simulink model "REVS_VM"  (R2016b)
settings: Solver=ode3  StartTime=REVS.sim_start_time_secs  StopTime=Inf  FixedStep=REVS.sim_step_time_secs  MaxStep=REVS.sim_step_time_secs  EnableMultiTasking=on
StopFcn:
  | postproc_datalog;
  | postproc_audit;
  | postproc_result;
model workspace (MATLAB code in the model file):
  other statements: REVS_setup_variants
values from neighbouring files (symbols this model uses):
  accessory = class_accessory_data    [class_test_data.m]
  battery = class_battery_data    [class_accessory_data.m]    (also in class_REVS_electric.m = class_REVS_battery)
  brake = struct(	'max_torque_Nm',[], 						'proportion_norm',1.0, 						'inertia_kgm2',0.0)    [class_REVS_drive_axle.m]
  engine = class_engine_data    [class_test_data.m]
  final_drive = struct(	'gear_ratio',[], 								'efficiency_norm',[], 								'inertia_kgm2',[] )    [class_REVS_drive_axle.m]
  gear = class_REVS_gearbox    [class_REVS_AT_transmission.m]
  tire = struct(	'radius_m',[], 						'rolling_resistance_coefficient',0, 						'vehicle_weight_norm',1.0,  						'wheel_slip_torque_Nm',[],  						'inertia_kgm2',0.0)    [class_REVS_drive_axle.m]
  torque_converter = class_REVS_torque_converter    [class_REVS_AT_transmission.m]
  transmission = class_transmission_data    [class_test_data.m]
  vehicle = class_vehicle_data    [class_test_data.m]
undefined symbols (not defined in the file or in its folder): alternator, ambient, controls, convert, DelayTimeSecs, drive_cycle, driver, electric, gear_strategy, InitialCondition, InitialValue, LoadSource, LookupStructure, MultiplyPosInputs, Normalize, NumPhases, REVS, SpeedSource, starter, tableshift, UpperSaturationLimit, Value, VerboseLevel, VerboseSignal
libraries: simulink x153
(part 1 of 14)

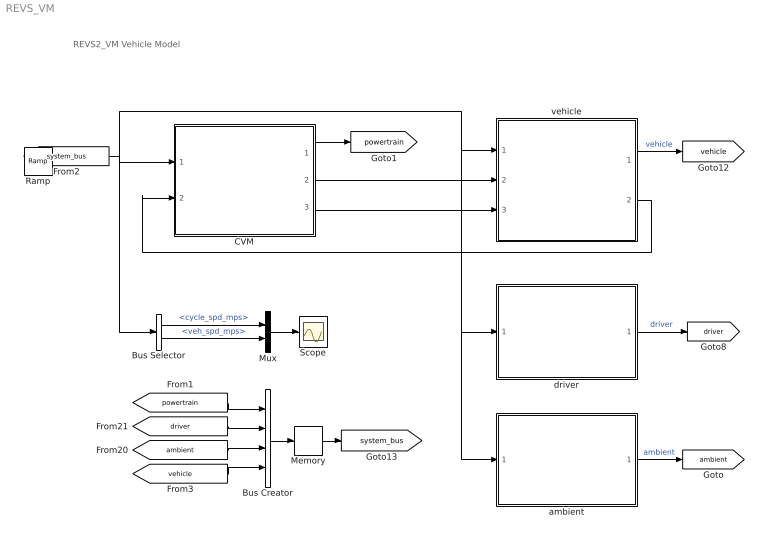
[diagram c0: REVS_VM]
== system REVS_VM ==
  note: REVS2_VM Vehicle Model
  Bus Creator : BusCreator  Inputs=4
  Bus Selector : BusSelector  OutputSignals=driver.cycle_spd_mps,vehicle.veh_spd_mps
  CVM : Subsystem  VariantControl=get_REVS_powertrain_type(REVS) == enum_powertrain_type.conventional
  Memory : Memory
  Mux : Mux  Inputs=2
  Scope : Scope
  ambient : Subsystem
  driver : Subsystem  VariantControl=variants_driver_MT
  vehicle : Subsystem
  Ramp : simulink/Sources/Ramp  IOType=siggen  slope=1  start=0  X0=0
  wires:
  vehicle/1(bus_out) -> [vehicle]  "vehicle"
  Bus Selector/1 -> Mux/1  "<cycle_spd_mps>"
  Bus Selector/2 -> Mux/2  "<veh_spd_mps>"
  Mux/1 -> Scope/1
  Bus Creator/1 -> Memory/1
  [driver] -> Bus Creator/2
  [ambient] -> Bus Creator/3
  Memory/1 -> [system_bus]
  [system_bus] -> CVM/1(system_bus), vehicle/1(system_bus), ambient/1(system_bus), driver/1(system_bus), Bus Selector/1
  [powertrain] -> Bus Creator/1
  [vehicle] -> Bus Creator/4
  vehicle/2(veh_spd_mps) -> CVM/2(veh_spd_mps)
  CVM/2(force_out_N) -> vehicle/2(force_in_N)
  CVM/3(mass_out_kg) -> vehicle/3(mass_in_kg)
  CVM/1(bus_out) -> [powertrain]
  ambient/1(bus_out) -> [ambient]  "ambient"
  driver/1(bus_out) -> [driver]  "driver"

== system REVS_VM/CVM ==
  note: ALPHA_CVM Conventional Vehicle Model
  system_bus : Inport
  veh_spd_mps : Inport  Port=2
  ALPHA CVM electric & accessories : Subsystem  VariantControl=variants_electric_ALPHA
  Bus Creator1 : BusCreator  Inputs=4
  CVM control : Subsystem
  automatic transmission system : Subsystem  VariantControl=get_REVS_transmission_type(transmission) == enum_transmission_type.automatic
  engine : Subsystem  Variant=on
  one axle drive : Subsystem  VariantControl=vehicle_driveline_type == enum_driveline_type.one_axle_drive
  bus_out : Outport
  force_out_N : Outport  Port=2
  mass_out_kg : Outport  Port=3
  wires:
  one axle drive/2(mass_out_kg) -> mass_out_kg/1
  one axle drive/1(force_out_N) -> force_out_N/1
  veh_spd_mps/1 -> one axle drive/4(spd_out_mps)
  system_bus/1 -> one axle drive/1(system_bus), automatic transmission system/1(system_bus), ALPHA CVM electric & accessories/1(system_bus), engine/1(system_bus), CVM control/1(system_bus)
  [trans] -> Bus Creator1/3
  [engine] -> Bus Creator1/2
  [control] -> Bus Creator1/1
  [electric] -> Bus Creator1/4
  Bus Creator1/1 -> bus_out/1  "powertrain"
  engine/2(eng_trq_Nm) -> automatic transmission system/2(trq_in_Nm)
  automatic transmission system/1(bus_out) -> [trans]
  engine/1(bus_out) -> [engine]
  automatic transmission system/2(trq_out_Nm) -> one axle drive/2(trq_in_Nm)
  ALPHA CVM electric & accessories/1(bus_out) -> [electric]
  automatic transmission system/3(iner_out_kgm2) -> one axle drive/3(iner_in_kgm2)
  one axle drive/3(spd_in_radps) -> automatic transmission system/4(spd_out_radps)
  ALPHA CVM electric & accessories/3(iner_out_kgm2) -> engine/3(acc_iner_kgm2)
  engine/3(eng_iner_kgm2) -> automatic transmission system/3(iner_in_kgm2)
  automatic transmission system/4(spd_in_radps) -> engine/4(eng_spd_radps), ALPHA CVM electric & accessories/2(spd_in_radps)
  ALPHA CVM electric & accessories/2(trq_out_Nm) -> engine/2(acc_trq_Nm)
  CVM control/1(bus_out) -> [control]

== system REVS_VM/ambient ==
  system_bus : Inport
  1-D Lookup Table : Lookup_n-D  NumberOfTableDimensions=1  BreakpointsForDimension1=drive_cycle.grade_dist_m  IndexSearchMethod=Linear search  BeginIndexSearchUsingPreviousIndexResult=on  Table=drive_cycle.grade_pct  ExtrapMethod=Clip  UseLastTableValue=on  RndMeth=Simplest
  Bus Creator : BusCreator  Inputs=2
  Bus Selector : BusSelector  OutputSignals=signal4.veh_dist_m
  Constant : Constant  Value=ambient.temperature_degC
  Time Logging : Subsystem
  datalog cycle grade : Subsystem
  bus_out : Outport
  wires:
  Constant/1 -> Bus Creator/2  "temp_degC"
  1-D Lookup Table/1 -> datalog cycle grade/1(Var), Bus Creator/1  "drive_cycle_grade_pct"
  Bus Creator/1 -> bus_out/1  "ambient"
  system_bus/1 -> Bus Selector/1
  Bus Selector/1 -> 1-D Lookup Table/1  "<veh_dist_m>"

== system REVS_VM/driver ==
  system_bus : Inport
  > 0 : Saturate  UpperLimit=Inf  LowerLimit=0
  Bus Creator1 : BusCreator  Inputs=8
  Compare To Zero : simulink/Logic and Bit Operations/Compare To Zero  relop=>  OutDataTypeStr=boolean
  Product : Product
  Product1 : Product
  closed loop driver : Subsystem
  cycle position : Subsystem
  datalog driver acl : Subsystem
  datalog driver brk : Subsystem
  drive cycle lookups : Subsystem
  bus_out : Outport
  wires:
  > 0/1 -> Bus Creator1/5  "cycle_spd_mps"
  drive cycle lookups/6(cycle_phase) -> Bus Creator1/7  "cycle_phase_num"
  drive cycle lookups/1(veh_spd_des_mps) -> closed loop driver/2(veh_spd_des_mps), > 0/1
  drive cycle lookups/2(future_veh_spd_des_mps) -> closed loop driver/3(future_veh_spd_des_mps)
  system_bus/1 -> cycle position/1(system_bus), closed loop driver/1(system_bus)
  Bus Creator1/1 -> bus_out/1  "driver"
  closed loop driver/1(acl_pedal_norm) -> Product/1
  closed loop driver/2(brk_pedal_norm) -> Product1/1
  drive cycle lookups/4(driver_key_pos) -> Bus Creator1/4  "driver_ign_keyon"
  Product/1 -> datalog driver acl/1(Var), Bus Creator1/1  "driver_acl_norm"
  Product1/1 -> datalog driver brk/1(Var), Bus Creator1/2  "driver_brk_norm"
  drive cycle lookups/3(driver_in_gear) -> Product/2, Product1/2, Bus Creator1/3  "driver_in_gear"
  cycle position/1(cycle_position_secs) -> Bus Creator1/8, drive cycle lookups/1(cycle_position_secs)  "cycle_pos_secs"
  drive cycle lookups/5(anticipate_veh_spd_des_mps) -> Compare To Zero/1
  Compare To Zero/1 -> Bus Creator1/6  "accel_anticipate_bool"

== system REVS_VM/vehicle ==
  system_bus : Inport
  force_in_N : Inport  Port=2
  mass_in_kg : Inport  Port=3
  Bus Creator : BusCreator  Inputs=2
  vehicle net force : Subsystem  VariantControl=vehicle_use_abc_roadload == true
  vehicle speed integrator : Subsystem
  bus_out : Outport
  veh_spd_mps : Outport  Port=2
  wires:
  Bus Creator/1 -> bus_out/1  "vehicle"
  system_bus/1 -> vehicle net force/1(system_bus), vehicle speed integrator/1(system_bus)
  force_in_N/1 -> vehicle net force/2(force_in_N)
  mass_in_kg/1 -> vehicle speed integrator/3(mass_in_kg)
  vehicle net force/1(force_out_N) -> vehicle speed integrator/2(force_out_N)
  vehicle speed integrator/1(veh_spd_mps) -> Bus Creator/1, veh_spd_mps/1, vehicle net force/3(chs_spd_mps)  "veh_spd_mps"
  vehicle speed integrator/2(veh_dist_m) -> Bus Creator/2  "veh_dist_m"

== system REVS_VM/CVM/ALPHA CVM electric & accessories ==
  system_bus : Inport
  spd_in_radps : Inport  Port=2
  Bus Creator : BusCreator  Inputs=2
  CVM accessories : Subsystem  VariantControl=variants_electric_ALPHA
  CVM electric : Subsystem  VariantControl=variants_electric_ALPHA
  Sum2 : Sum
  Sum6 : Sum
  bus_out : Outport
  trq_out_Nm : Outport  Port=2
  iner_out_kgm2 : Outport  Port=3
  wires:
  spd_in_radps/1 -> CVM accessories/2(spd_in_radps), CVM electric/2(spd_in_radps)
  Bus Creator/1 -> bus_out/1
  system_bus/1 -> CVM electric/1(system_bus), CVM accessories/1(system_bus)
  Sum6/1 -> iner_out_kgm2/1
  Sum2/1 -> trq_out_Nm/1
  CVM accessories/4(curr_out_A) -> CVM electric/3(curr_in_A)
  CVM electric/3(iner_out_kgm2) -> Sum6/1
  CVM electric/1(bus_out) -> Bus Creator/1  "elec"
  CVM accessories/1(bus_out) -> Bus Creator/2  "accy"
  CVM electric/4(volt_out_V) -> CVM accessories/3(voltage_V)
  CVM accessories/3(iner_out_kgm2) -> Sum6/2
  CVM accessories/2(trq_out_Nm) -> Sum2/2
  CVM electric/2(trq_out_Nm) -> Sum2/1

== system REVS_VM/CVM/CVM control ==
  system_bus : Inport
  Bus Creator : BusCreator  Inputs=1
  start stop logic : Subsystem
  bus_out : Outport
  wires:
  start stop logic/1(engine_on) -> Bus Creator/1  "ctrl_eng_on"
  system_bus/1 -> start stop logic/1(system_bus)
  Bus Creator/1 -> bus_out/1  "control"

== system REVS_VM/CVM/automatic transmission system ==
  system_bus : Inport
  trq_in_Nm : Inport  Port=2
  iner_in_kgm2 : Inport  Port=3
  spd_out_radps : Inport  Port=4
  Bus Creator : BusCreator  Inputs=4
  automatic trans control : Subsystem  VariantControl=variants_trans_control_default
  automatic transmission core : Subsystem  VariantControl=variants_trans_automatic
  result work : Subsystem
  thermal model : Subsystem  Variant=on
  to datalog : Subsystem
  to datalog1 : Subsystem
  to datalog2 : Subsystem
  torque converter : Subsystem
  bus_out : Outport
  trq_out_Nm : Outport  Port=2
  iner_out_kgm2 : Outport  Port=3
  spd_in_radps : Outport  Port=4
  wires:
  thermal model/1(thermal_bus) -> Bus Creator/2  "therm"
  automatic transmission core/4(spd_in_radps) -> torque converter/4(spd_out_radps)
  torque converter/4(spd_in_radps) -> spd_in_radps/1
  spd_out_radps/1 -> to datalog2/1(Var), result work/2(speed_radps), automatic transmission core/4(spd_out_radps)  "trans_spd_out_radps"
  torque converter/3(iner_out_kgm2) -> automatic transmission core/3(iner_in_kgm2)
  torque converter/2(trq_out_Nm) -> automatic transmission core/2(trq_in_Nm)
  iner_in_kgm2/1 -> torque converter/3(iner_in_kgm2)
  trq_in_Nm/1 -> torque converter/2(trq_in_Nm)
  automatic transmission core/3(iner_out_kgm2) -> iner_out_kgm2/1, to datalog1/1(Var), result work/3(upstream_iner_kgm2)
  automatic transmission core/2(trq_out_Nm) -> to datalog/1(Var), result work/1(torque_Nm), trq_out_Nm/1
  automatic transmission core/1(bus_out) -> Bus Creator/4  "core"
  automatic trans control/1(bus_out) -> Bus Creator/1  "ctrl"
  system_bus/1 -> automatic trans control/1(system_bus), thermal model/1(system_bus)
  Bus Creator/1 -> bus_out/1, torque converter/1(trans_bus), automatic transmission core/1(trans_bus)  "trans"
  torque converter/1(bus_out) -> Bus Creator/3  "trq_conv"

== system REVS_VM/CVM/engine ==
  note: 1) Only subsystems can be added as variant choices at this level 2) Blocks cannot be connected at this level as connectivity is automatically determined at simulation, based on the active variant
  system_bus : Inport
  acc_trq_Nm : Inport  Port=2
  acc_iner_kgm2 : Inport  Port=3
  eng_spd_radps : Inport  Port=4
  legacy engine : Subsystem  VariantControl=get_REVS_engine_model_type(engine) == enum_engine_model_type.legacy
  new engine : Subsystem  VariantControl=get_REVS_engine_model_type(engine) == enum_engine_model_type.current
  bus_out : Outport
  eng_trq_Nm : Outport  Port=2
  eng_iner_kgm2 : Outport  Port=3

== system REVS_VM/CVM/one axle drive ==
  system_bus : Inport
  trq_in_Nm : Inport  Port=2
  iner_in_kgm2 : Inport  Port=3
  spd_out_mps : Inport  Port=4
  Drive  Axle : Subsystem
  force_out_N : Outport
  mass_out_kg : Outport  Port=2
  spd_in_radps : Outport  Port=3
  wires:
  spd_out_mps/1 -> Drive  Axle/4(spd_out_mps)
  iner_in_kgm2/1 -> Drive  Axle/3(iner_in_kgm2)
  trq_in_Nm/1 -> Drive  Axle/2(trq_in_Nm)
  system_bus/1 -> Drive  Axle/1(system bus)
  Drive  Axle/3(spd_in_radps) -> spd_in_radps/1
  Drive  Axle/2(mass_out_kg) -> mass_out_kg/1
  Drive  Axle/1(force_out_N) -> force_out_N/1

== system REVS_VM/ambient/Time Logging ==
  Align to cycle position : Bias  Bias=-5
  Clock : Clock
  Constant : Constant  Value=REVS.verbose >= 0
  time : Subsystem
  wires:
  Align to cycle position/1 -> time/1("time ")
  Constant/1 -> time/Enable
  Clock/1 -> Align to cycle position/1

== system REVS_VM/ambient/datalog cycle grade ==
  Var : Inport
  Constant : Constant  Value=VerboseSignal
  Constant1 : Constant  Value=VerboseLevel
  Relational Operator : RelationalOperator  OutDataTypeStr=boolean  ZeroCross=off
  Subsystem : Subsystem
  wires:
  Constant1/1 -> Relational Operator/2
  Constant/1 -> Relational Operator/1
  Relational Operator/1 -> Subsystem/Enable
  Var/1 -> Subsystem/1(In1)

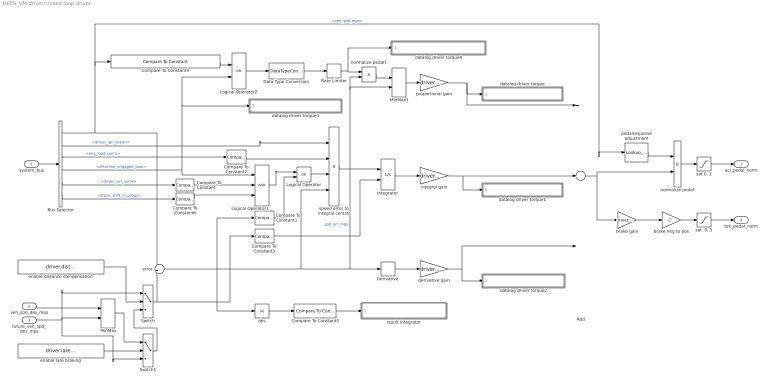
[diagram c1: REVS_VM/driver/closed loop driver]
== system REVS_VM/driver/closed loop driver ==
  system_bus : Inport
  veh_spd_des_mps : Inport  Port=2
  future_veh_spd_des_mps : Inport  Port=3
  Add : Sum  Inputs=+++
  Bus Selector : BusSelector  OutputSignals=vehicle.veh_spd_mps,driver.driver_ign_keyon,powertrain.engine.eng_load_norm,powertrain.trans.ctrl.core_ctl.driveline_engaged_bool,driver.driver_acl_norm,powertrain.trans.ctrl.core_ctl.trans_shift_in_prog
  Compare To Constant : simulink/Logic and Bit Operations/Compare To Constant  relop=<  const=1  OutDataTypeStr=boolean  ZeroCross=off
  Compare To Constant1 : simulink/Logic and Bit Operations/Compare To Constant  relop=<  const=0  OutDataTypeStr=boolean  ZeroCross=off
  Compare To Constant2 : simulink/Logic and Bit Operations/Compare To Constant  relop=<  const=0.99  OutDataTypeStr=boolean  ZeroCross=off
  Compare To Constant3 : simulink/Logic and Bit Operations/Compare To Constant  relop=<=  const=0  OutDataTypeStr=boolean  ZeroCross=off
  Compare To Constant4 : simulink/Logic and Bit Operations/Compare To Constant  relop=<  const=driver.proportional_fade_in_min_speed_mps  OutDataTypeStr=boolean  ZeroCross=off
  Compare To Constant5 : simulink/Logic and Bit Operations/Compare To Constant  relop=>  const=2*convert.mph2mps  OutDataTypeStr=boolean  ZeroCross=off
  Compare To Constant6 : simulink/Logic and Bit Operations/Compare To Constant  relop===  const=0  OutDataTypeStr=boolean  ZeroCross=off
  Data Type Conversion : DataTypeConversion
  Derivative : Derivative
  Integrator : Integrator  ExternalReset=level  LimitOutput=on  LowerSaturationLimit=0  ZeroCross=off
  Logical Operator : Logic  Operator=OR  AllPortsSameDT=off  OutDataTypeStr=boolean
  Logical Operator1 : Logic  Inputs=3  AllPortsSameDT=off  OutDataTypeStr=boolean
  Logical Operator2 : Logic  Operator=OR  AllPortsSameDT=off  OutDataTypeStr=boolean
  MinMax : MinMax  Function=max  Inputs=2  ZeroCross=off
  MinMax1 : MinMax  Inputs=2  ZeroCross=off
  Rate Limiter : RateLimiter  RisingSlewLimit=1/driver.proportional_fade_in_secs  FallingSlewLimit=-inf  LinearizeAsGain=off
  Switch : Switch  Criteria=u2 ~= 0  ZeroCross=off
  Switch1 : Switch  Criteria=u2 ~= 0  ZeroCross=off
  abs : Abs
  brake gain : Gain  Gain=driver.brake_gain_norm
  brake neg to pos : Gain  Gain=-1
  datalog driver torque : Subsystem
  datalog driver torque1 : Subsystem
  datalog driver torque2 : Subsystem
  datalog driver torque3 : Subsystem
  datalog driver torque4 : Subsystem
  derivative gain : Gain  Gain=driver.Kd
  enable distance compensation : Constant  Value=driver.distance_compensate_enable
  enable late braking : Constant  Value=driver.late_braking
  error : Sum  Inputs=-+
  integral gain : Gain  Gain=driver.Ki/100
  normalize pedal : Product  Inputs=**
  normalize pedal1 : Product  Inputs=**
  pedalresponse adjustment : Lookup_n-D  NumberOfTableDimensions=1  BreakpointsForDimension1=driver.accel_pedal_response_speed_mps  IndexSearchMethod=Linear search  BeginIndexSearchUsingPreviousIndexResult=on  Table=driver.accel_pedal_response_norm  ExtrapMethod=Clip  UseLastTableValue=on  RndMeth=Simplest
  proportional gain : Gain  Description=1.3 factor converts REVS1 Kp to REVS2 Kp, more or less  RequirementInfo={} %GIDa_c10416ae_7039_4e6e_8729_c37e926f399b  Gain=driver.Kp * 1.3
  result integrator : Subsystem
  sat  0..1 : Saturate  UpperLimit=1  LowerLimit=0  ZeroCross=off
  sat 0..1 : Saturate  UpperLimit=1  LowerLimit=0  ZeroCross=off
  speed error to integral control : Product  Inputs=4
  acl_pedal_norm : Outport
  brk_pedal_norm : Outport  Port=2
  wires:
  Switch1/1 -> Switch/3
  enable late braking/1 -> Switch1/2
  brake neg to pos/1 -> sat  0..1/1
  abs/1 -> Compare To Constant5/1
  Compare To Constant5/1 -> result integrator/1(in)
  Data Type Conversion/1 -> Rate Limiter/1
  MinMax1/1 -> proportional gain/1
  Rate Limiter/1 -> normalize pedal1/1, datalog driver torque4/1(Var)
  Compare To Constant4/1 -> Logical Operator2/1
  Logical Operator1/1 -> Logical Operator/1
  Compare To Constant3/1 -> Integrator/2
  Switch/1 -> error/2, Compare To Constant3/1
  Compare To Constant2/1 -> speed error to integral control/2
  Bus Selector/3 -> Compare To Constant2/1  "<eng_load_norm>"
  Logical Operator/1 -> speed error to integral control/3
  Compare To Constant1/1 -> Logical Operator/2
  Compare To Constant/1 -> Logical Operator1/2
  Bus Selector/5 -> Compare To Constant/1  "<driver_acl_norm>"
  Integrator/1 -> integral gain/1
  Derivative/1 -> derivative gain/1
  veh_spd_des_mps/1 -> MinMax/1
  system_bus/1 -> Bus Selector/1
  speed error to integral control/1 -> Integrator/1
  error/1 -> MinMax1/2, normalize pedal1/2, Derivative/1, speed error to integral control/4, abs/1, Compare To Constant1/1  "spd_err_mps"
  integral gain/1 -> Add/2, datalog driver torque1/1(Var)
  derivative gain/1 -> Add/3, datalog driver torque2/1(Var)
  Bus Selector/4 -> Logical Operator2/2, datalog driver torque3/1(Var), Logical Operator1/1  "<driveline_engaged_bool>"
  Bus Selector/1 -> pedalresponse adjustment/1, Compare To Constant4/1, error/1  "<veh_spd_mps>"
  future_veh_spd_des_mps/1 -> Switch/1, MinMax/2, Switch1/3
  enable distance compensation/1 -> Switch/2
  MinMax/1 -> Switch1/1
  Bus Selector/2 -> speed error to integral control/1  "<driver_ign_keyon>"
  pedalresponse adjustment/1 -> normalize pedal/1
  normalize pedal/1 -> sat 0..1/1
  Add/1 -> brake gain/1, normalize pedal/2
  sat 0..1/1 -> acl_pedal_norm/1
  sat  0..1/1 -> brk_pedal_norm/1
  brake gain/1 -> brake neg to pos/1
  proportional gain/1 -> datalog driver torque/1(Var), Add/1
  normalize pedal1/1 -> MinMax1/1
  Logical Operator2/1 -> Data Type Conversion/1
  Compare To Constant6/1 -> Logical Operator1/3
  Bus Selector/6 -> Compare To Constant6/1  "<trans_shift_in_prog>"

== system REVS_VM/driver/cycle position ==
  system_bus : Inport
  Bias : Bias  Bias=eps
  Bias1 : Bias  Bias=eps
  Bus Selector : BusSelector  OutputSignals=vehicle.veh_spd_mps,driver.cycle_spd_mps,driver.driver_in_gear
  Compare To Constant : simulink/Logic and Bit Operations/Compare To Constant  relop=>=  const=1.0  OutDataTypeStr=boolean  ZeroCross=off
  Compare To Constant1 : simulink/Logic and Bit Operations/Compare To Constant  relop=<=  const=1e-9  OutDataTypeStr=boolean
  Divide : Product  Inputs=*/
  Integrator : Integrator  InitialCondition=-5
  Sum3 : Sum  Inputs=++|
  Sum4 : Sum  Inputs=-+|
  enable distance compensation : Constant  Value=driver.distance_compensate_enable
  mult : Product  Inputs=4
  time delay fault : Subsystem
  unity : Constant
  cycle_position_secs : Outport
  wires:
  Integrator/1 -> cycle_position_secs/1
  Bias1/1 -> Divide/1
  Bias/1 -> Divide/2
  Sum3/1 -> Integrator/1, Compare To Constant1/1
  Divide/1 -> Sum4/2
  unity/1 -> Sum4/1, Sum3/1
  Compare To Constant/1 -> mult/2
  Sum4/1 -> mult/1
  Bus Selector/1 -> Bias1/1  "<veh_spd_mps>"
  system_bus/1 -> Bus Selector/1
  Bus Selector/2 -> Compare To Constant/1, Bias/1  "<cycle_spd_mps>"
  enable distance compensation/1 -> mult/3
  mult/1 -> Sum3/2
  Compare To Constant1/1 -> time delay fault/1(" condition")
  Bus Selector/3 -> mult/4  "<driver_in_gear>"

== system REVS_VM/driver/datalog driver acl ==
  Var : Inport
  Constant : Constant  Value=VerboseSignal
  Constant1 : Constant  Value=VerboseLevel
  Relational Operator : RelationalOperator  OutDataTypeStr=boolean  ZeroCross=off
  Subsystem : Subsystem
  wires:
  Constant1/1 -> Relational Operator/2
  Constant/1 -> Relational Operator/1
  Relational Operator/1 -> Subsystem/Enable
  Var/1 -> Subsystem/1(In1)

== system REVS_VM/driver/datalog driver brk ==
  Var : Inport
  Constant : Constant  Value=VerboseSignal
  Constant1 : Constant  Value=VerboseLevel
  Relational Operator : RelationalOperator  OutDataTypeStr=boolean  ZeroCross=off
  Subsystem : Subsystem
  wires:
  Constant1/1 -> Relational Operator/2
  Constant/1 -> Relational Operator/1
  Relational Operator/1 -> Subsystem/Enable
  Var/1 -> Subsystem/1(In1)

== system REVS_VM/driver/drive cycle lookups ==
  cycle_position_secs : Inport
  Compare To Zero : simulink/Logic and Bit Operations/Compare To Zero  relop=<=  OutDataTypeStr=uint8  ZeroCross=off
  Compare To Zero1 : simulink/Logic and Bit Operations/Compare To Zero  relop=<=  OutDataTypeStr=uint8  ZeroCross=off
  Compare To Zero2 : simulink/Logic and Bit Operations/Compare To Zero  relop=>=  OutDataTypeStr=boolean
  Constant : Constant  Value=driver.lookahead_secs
  Constant2 : Constant  Value=drive_cycle.sample_start_enable
  Data Type Conversion : DataTypeConversion
  Data Type Conversion1 : DataTypeConversion
  Gain : Gain  Gain=0.1
  Gain1 : Gain  Gain=0.1
  Logical Operator : Logic  Operator=OR  AllPortsSameDT=off  OutDataTypeStr=boolean
  Product : Product
  Stop Simulation : Stop
  Sum : Sum  Inputs=++|
  Sum1 : Sum  Inputs=|+-
  Sum2 : Sum  Inputs=|+-
  Sum4 : Sum  Inputs=++|
  datalog desired speed : Subsystem
  datalog drive cycle phase : Subsystem
  drive cycle : Lookup_n-D  NumberOfTableDimensions=1  BreakpointsForDimension1=drive_cycle.cycle_time  IndexSearchMethod=Linear search  BeginIndexSearchUsingPreviousIndexResult=on  Table=drive_cycle.cycle_speed_mps  ExtrapMethod=Clip  UseLastTableValue=on  RndMeth=Simplest  MaximumIndicesForEachDimension=1e5
  drive cycle ignition : Lookup_n-D  NumberOfTableDimensions=1  BreakpointsForDimension1=drive_cycle.ignition_time  IndexSearchMethod=Linear search  BeginIndexSearchUsingPreviousIndexResult=on  Table=drive_cycle.ignition  InterpMethod=Flat  ExtrapMethod=Clip  UseLastTableValue=on  RndMeth=Simplest  MaximumIndicesForEachDimension=1e5
  drive cycle in gear : Lookup_n-D  NumberOfTableDimensions=1  BreakpointsForDimension1=drive_cycle.in_gear_time  IndexSearchMethod=Linear search  BeginIndexSearchUsingPreviousIndexResult=on  Table=drive_cycle.in_gear  InterpMethod=Flat  ExtrapMethod=Clip  UseLastTableValue=on  RndMeth=Simplest  MaximumIndicesForEachDimension=1e5
  drive cycle phase : Lookup_n-D  NumberOfTableDimensions=1  BreakpointsForDimension1=drive_cycle.phase_time  IndexSearchMethod=Linear search  BeginIndexSearchUsingPreviousIndexResult=on  Table=drive_cycle.phase  InterpMethod=Flat  ExtrapMethod=Clip  UseLastTableValue=on  RndMeth=Simplest  MaximumIndicesForEachDimension=1e5
  end of cycle : simulink/Logic and Bit Operations/Compare To Constant  relop=>=  const=drive_cycle.cycle_time(end)  OutDataTypeStr=boolean
  future drive cycle : Lookup_n-D  NumberOfTableDimensions=1  BreakpointsForDimension1=drive_cycle.cycle_time  IndexSearchMethod=Linear search  BeginIndexSearchUsingPreviousIndexResult=on  Table=drive_cycle.cycle_speed_mps  ExtrapMethod=Clip  UseLastTableValue=on  RndMeth=Simplest  MaximumIndicesForEachDimension=1e5
  future drive cycle1 : Lookup_n-D  NumberOfTableDimensions=1  BreakpointsForDimension1=drive_cycle.cycle_time  IndexSearchMethod=Linear search  BeginIndexSearchUsingPreviousIndexResult=on  Table=drive_cycle.cycle_speed_mps  ExtrapMethod=Clip  UseLastTableValue=on  RndMeth=Simplest  MaximumIndicesForEachDimension=1e5
  result integrator : Subsystem
  result phase input : Subsystem
  start anticipate secs : Constant  Value=driver.launch_anticipate_secs
  veh_spd_des_mps : Outport
  future_veh_spd_des_mps : Outport  Port=2
  driver_in_gear : Outport  Port=3
  driver_key_pos : Outport  Port=4
  anticipate_veh_spd_des_mps : Outport  Port=5
  cycle_phase : Outport  Port=6
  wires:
  Data Type Conversion1/1 -> Gain1/1
  Data Type Conversion/1 -> Gain/1
  Gain1/1 -> Sum2/2
  Gain/1 -> Sum1/2
  Compare To Zero1/1 -> Data Type Conversion1/1
  Compare To Zero/1 -> Data Type Conversion/1
  Sum2/1 -> future_veh_spd_des_mps/1
  Sum1/1 -> veh_spd_des_mps/1
  Sum/1 -> future drive cycle/1
  future drive cycle/1 -> Sum2/1, Compare To Zero1/1
  drive cycle/1 -> datalog desired speed/1(Var), result integrator/1(in), Sum1/1, Compare To Zero/1
  Constant/1 -> Sum/1
  drive cycle in gear/1 -> driver_in_gear/1  "driver_in_gear"
  end of cycle/1 -> Stop Simulation/1
  drive cycle phase/1 -> Product/1
  Product/1 -> datalog drive cycle phase/1(Var), result phase input/1(phase), cycle_phase/1
  Compare To Zero2/1 -> Logical Operator/1
  Logical Operator/1 -> Product/2
  Constant2/1 -> Logical Operator/2
  drive cycle ignition/1 -> driver_key_pos/1
  Sum4/1 -> future drive cycle1/1
  start anticipate secs/1 -> Sum4/2
  cycle_position_secs/1 -> end of cycle/1, drive cycle/1, Sum/2, Compare To Zero2/1, Sum4/1, drive cycle ignition/1, drive cycle phase/1, drive cycle in gear/1
  future drive cycle1/1 -> anticipate_veh_spd_des_mps/1

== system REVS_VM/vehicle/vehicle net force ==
  system_bus : Inport
  force_in_N : Inport  Port=2
  chs_spd_mps : Inport  Port=3
  Compare To Zero : simulink/Logic and Bit Operations/Compare To Zero  relop===  OutDataTypeStr=boolean  ZeroCross=off
  Compare To Zero1 : simulink/Logic and Bit Operations/Compare To Zero  relop=~=  OutDataTypeStr=boolean  ZeroCross=off
  Mech E&P N mps0 : Subsystem
  Mech E&P N mps2 : Subsystem
  Mech E&P N mps3 : Subsystem
  Mech E&P N mps4 : Subsystem
  Product : Product
  Product1 : Product
  Sign1 : Gain  Gain=-1
  Sign2 : Gain  Gain=-1
  Sign3 : Gain  Gain=-1
  aerodynamic drag : Subsystem
  const : Constant  Value=vehicle.use_abc_roadload
  drag forces : Sum  Inputs=+++
  gradient force : Subsystem
  road load by ABC : Subsystem
  total force : Sum  Inputs=++|
  zero : Constant  Value=0
  force_out_N : Outport
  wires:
  system_bus/1 -> gradient force/1(system_bus), road load by ABC/1(system_bus)
  const/1 -> Compare To Zero1/1, Compare To Zero/1
  Compare To Zero/1 -> Product1/1
  Compare To Zero1/1 -> Product/2
  Sign3/1 -> Product1/2
  Sign2/1 -> Product/1
  chs_spd_mps/1 -> Mech E&P N mps3/2(spd_mps), Mech E&P N mps0/2(spd_mps), Mech E&P N mps2/2(spd_mps), Mech E&P N mps4/2(spd_mps), aerodynamic drag/1(veh_spd_mps), road load by ABC/2(veh_spd_mps)
  Product1/1 -> drag forces/3, Mech E&P N mps4/1(force_N)
  aerodynamic drag/1(aero_force_N) -> Sign3/1
  Product/1 -> drag forces/2, Mech E&P N mps2/1(force_N)
  road load by ABC/1(rdload_force_N) -> Sign2/1
  total force/1 -> force_out_N/1
  force_in_N/1 -> total force/1, Mech E&P N mps3/1(force_N)
  Sign1/1 -> drag forces/1, Mech E&P N mps0/1(force_N)
  drag forces/1 -> total force/2
  gradient force/1(grade_force_N) -> Sign1/1
  zero/1 -> Mech E&P N mps3/3(mass_kg)

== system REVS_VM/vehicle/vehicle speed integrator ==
  system_bus : Inport
  force_out_N : Inport  Port=2
  mass_in_kg : Inport  Port=3
  Compare To Constant : simulink/Logic and Bit Operations/Compare To Constant  relop=<=  const=0.1  OutDataTypeStr=boolean
  Dynamic Vehicle Mass (kg) : Constant  Value=vehicle.mass_dynamic_kg
  Integrator : Integrator  LimitOutput=on  UpperSaturationLimit=Inf  LowerSaturationLimit=0
  Integrator1 : Integrator  LimitOutput=on  UpperSaturationLimit=Inf  LowerSaturationLimit=0  ZeroCross=off
  Mech E&P N mps2 : Subsystem
  Product : Product  Inputs=*/
  Sum : Sum  Inputs=2
  Sum1 : Sum  Inputs=2
  dynamic lookup : Subsystem
  result integrator : Subsystem
  result integrator1 : Subsystem
  to datalog : Subsystem
  to datalog1 : Subsystem
  to datalog2 : Subsystem
  veh_spd_mps : Outport
  veh_dist_m : Outport  Port=2
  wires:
  dynamic lookup/1(out) -> Sum1/1
  Sum1/1 -> Mech E&P N mps2/3(mass_kg), Sum/2
  system_bus/1 -> dynamic lookup/1(bus)
  Compare To Constant/1 -> result integrator1/1(in)
  Integrator1/1 -> veh_dist_m/1, to datalog2/1(Var)
  Sum/1 -> Product/2, to datalog/1(Var)
  mass_in_kg/1 -> Sum/1
  Dynamic Vehicle Mass (kg)/1 -> Sum1/2
  Integrator/1 -> veh_spd_mps/1, Integrator1/1, result integrator/1(in), Compare To Constant/1, Mech E&P N mps2/2(spd_mps), to datalog1/1(Var)
  Product/1 -> Integrator/1
  force_out_N/1 -> Mech E&P N mps2/1(force_N), Product/1

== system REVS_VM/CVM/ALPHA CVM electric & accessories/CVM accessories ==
  system_bus : Inport
  spd_in_radps : Inport  Port=2
  voltage_V : Inport  Port=3
  Elec E&P V A Standalone : Subsystem
  Mech E&P Nm radps : Subsystem
  Sum3 : Sum  Inputs=++++
  Sum4 : Sum  Inputs=++++
  Sum5 : Sum  Inputs=++++
  air conditioning : Subsystem
  fan loss : Subsystem
  generic loss : Subsystem
  power steering : Subsystem
  bus_out : Outport
  trq_out_Nm : Outport  Port=2
  iner_out_kgm2 : Outport  Port=3
  curr_out_A : Outport  Port=4
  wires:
  Sum5/1 -> Elec E&P V A Standalone/2(curr_A), curr_out_A/1
  fan loss/3(inertia_kgm2) -> Sum3/4
  air conditioning/3(inertia_kgm2) -> Sum3/3
  power steering/3(inertia_kgm2) -> Sum3/2
  fan loss/2(torque_Nm) -> Sum4/4
  air conditioning/2(torque_Nm) -> Sum4/3
  power steering/2(torque_Nm) -> Sum4/2
  spd_in_radps/1 -> Mech E&P Nm radps/2(spd_radps), generic loss/3(speed_radps), power steering/3(speed_radps), air conditioning/3(speed_radps), fan loss/3(speed_radps)
  fan loss/1(curr_in_A) -> Sum5/4
  air conditioning/1(curr_in_A) -> Sum5/3
  power steering/1(curr_in_A) -> Sum5/2
  generic loss/1(curr_in_A) -> Sum5/1
  voltage_V/1 -> Elec E&P V A Standalone/1(volts_V), fan loss/2(voltage_volts), air conditioning/2(voltage_volts), power steering/2(voltage_volts), generic loss/2(voltage_volts)
  system_bus/1 -> generic loss/1(system_bus), power steering/1(system_bus), air conditioning/1(system_bus), fan loss/1(system_bus)
  Sum3/1 -> iner_out_kgm2/1
  Sum4/1 -> Mech E&P Nm radps/1(trq_Nm), trq_out_Nm/1
  generic loss/3(inertia_kgm2) -> Sum3/1
  generic loss/2(torque_Nm) -> Sum4/1

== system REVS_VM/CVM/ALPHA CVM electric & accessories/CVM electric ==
  system_bus : Inport
  spd_in_radps : Inport  Port=2
  curr_in_A : Inport  Port=3
  Sum1 : Sum  Inputs=+++
  Sum2 : Sum  Inputs=|++
  Sum3 : Sum  Inputs=++|
  alternator : Subsystem
  battery : Subsystem
  starter motor (simple) : Subsystem
  bus_out : Outport
  trq_out_Nm : Outport  Port=2
  iner_out_kgm2 : Outport  Port=3
  volt_out_V : Outport  Port=4
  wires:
  curr_in_A/1 -> Sum1/3
  Sum1/1 -> battery/2(curr_out_A)
  alternator/3(curr_out_A) -> Sum1/2
  starter motor (simple)/3(curr_out_A) -> Sum1/1
  battery/1(bus_out) -> bus_out/1
  starter motor (simple)/1(trq_out_Nm) -> Sum2/1
  alternator/1(trq_out_Nm) -> Sum2/2
  starter motor (simple)/2(iner_out_kgm2) -> Sum3/1
  alternator/2(iner_out_kgm2) -> Sum3/2
  battery/2(volts_out_V) -> alternator/2(batt_volts_V), starter motor (simple)/2(batt_volts_V), volt_out_V/1
  system_bus/1 -> starter motor (simple)/1(system_bus), alternator/1(system_bus), battery/1(system_bus)
  Sum3/1 -> iner_out_kgm2/1
  Sum2/1 -> trq_out_Nm/1
  spd_in_radps/1 -> starter motor (simple)/3(spd_in_radps), alternator/3(spd_in_radps)

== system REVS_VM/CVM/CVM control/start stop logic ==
  system_bus : Inport
  Bus Selector : BusSelector  OutputSignals=driver.driver_ign_keyon,vehicle.veh_spd_mps,driver.accel_anticipate_bool
  Compare To Constant : simulink/Logic and Bit Operations/Compare To Constant  relop=>=  const=controls.stop_delay_secs  OutDataTypeStr=boolean
  Logical Operator2 : Logic  Operator=NAND  Inputs=4  AllPortsSameDT=off  OutDataTypeStr=boolean
  Logical Operator3 : Logic  Operator=NOT  AllPortsSameDT=off  OutDataTypeStr=boolean
  Logical Operator4 : Logic  AllPortsSameDT=off  OutDataTypeStr=boolean
  stop start enable : Constant  Value=controls.start_stop_enable
  stop time : Subsystem
  stopped speed : simulink/Logic and Bit Operations/Compare To Constant  relop=<=  const=0.1  OutDataTypeStr=boolean
  to datalog1 : Subsystem
  to datalog2 : Subsystem
  to datalog3 : Subsystem
  warmup condition : Subsystem
  engine_on : Outport
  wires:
  Bus Selector/1 -> Logical Operator4/1  "<driver_ign_keyon>"
  stop time/1(out) -> Compare To Constant/1
  stopped speed/1 -> stop time/1(bool)
  system_bus/1 -> Bus Selector/1, warmup condition/1(bus)
  warmup condition/1(out) -> Logical Operator2/3
  Bus Selector/3 -> Logical Operator3/1, to datalog1/1(Var)  "<accel_anticipate_bool>"
  stop start enable/1 -> Logical Operator2/4
  Logical Operator3/1 -> Logical Operator2/2
  Bus Selector/2 -> stopped speed/1  "<veh_spd_mps>"
  Compare To Constant/1 -> to datalog3/1(Var), Logical Operator2/1
  Logical Operator2/1 -> Logical Operator4/2
  Logical Operator4/1 -> to datalog2/1(Var), engine_on/1

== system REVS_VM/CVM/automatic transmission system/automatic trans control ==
  system_bus : Inport
  Bus Creator : BusCreator  Inputs=10
  Bus Selector1 : BusSelector  OutputSignals=powertrain.trans.core.gearbox.gb_curr_gear
  Bus Selector2 : BusSelector  OutputSignals=driver.driver_acl_norm
  Compare To Zero : simulink/Logic and Bit Operations/Compare To Zero  relop=>  OutDataTypeStr=boolean  ZeroCross=off
  Divide : Product  Inputs=**
  Logical Operator1 : Logic  Operator=NOT  AllPortsSameDT=off  OutDataTypeStr=boolean
  Saturation : Saturate  UpperLimit=1  LowerLimit=-1
  Sum : Sum  Inputs=+-
  auto neutral logic : Subsystem
  comp_iner_enable1 : Constant  Value=Inf
  driver acl to eng des acl : Gain
  gb curr gear to tans curr gear : Gain
  gear select : Subsystem  Variant=on
  line pressure control : Subsystem
  lockup select : Subsystem  Variant=on
  shift counter : Subsystem
  to datalog : Subsystem
  to datalog1 : Subsystem
  to datalog2 : Subsystem
  to datalog5 : Subsystem
  trans des eng spd : Constant  Value=0
  upshift inertia compensation : Subsystem
  bus_out : Outport
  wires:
  upshift inertia compensation/1(comp_iner_enable) -> Bus Creator/4  "eng_comp_iner_enable"
  Bus Selector2/1 -> driver acl to eng des acl/1  "<driver_acl_norm>"
  Bus Selector1/1 -> lockup select/1(gear_number), gb curr gear to tans curr gear/1  "<gb_curr_gear>"
  gb curr gear to tans curr gear/1 -> to datalog5/1(Var), Bus Creator/10, Sum/2  "trans_curr_gear"
  line pressure control/1(cmd_line_press_bar) -> to datalog2/1(Var), Bus Creator/8  "gb_line_press_bar"
  comp_iner_enable1/1 -> Bus Creator/7  "eng_des_load_limit_Nm"
  Divide/1 -> Bus Creator/1, Compare To Zero/1, Sum/1, shift counter/1(target_gear)  "gear_num"
  system_bus/1 -> line pressure control/1(system_bus), Bus Selector2/1, Bus Selector1/1, upshift inertia compensation/1(system_bus), gear select/1(system_bus), auto neutral logic/1(system_bus), lockup select/2(system_bus)
  Bus Creator/1 -> bus_out/1  "ctrl"
  lockup select/1(lockup_cmd) -> Bus Creator/3, to datalog/1(Var)  "tcc_lockup_cmd_bool"
  driver acl to eng des acl/1 -> Bus Creator/5  "eng_des_acl_norm"
  trans des eng spd/1 -> Bus Creator/6  "eng_des_spd_radps"
  Compare To Zero/1 -> Bus Creator/2  "driveline_engaged_bool"
  gear select/1(target_gear) -> to datalog1/1(Var), Divide/1
  auto neutral logic/1(auto_neutral_bool) -> Logical Operator1/1
  Logical Operator1/1 -> Divide/2
  Sum/1 -> Saturation/1
  Saturation/1 -> Bus Creator/9  "trans_shift_in_prog"

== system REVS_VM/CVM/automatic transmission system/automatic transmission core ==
  trans_bus : Inport
  trq_in_Nm : Inport  Port=2
  iner_in_kgm2 : Inport  Port=3
  spd_out_radps : Inport  Port=4
  Bus Creator : BusCreator  Inputs=3
  gearbox : Subsystem
  bus_out : Outport
  trq_out_Nm : Outport  Port=2
  iner_out_kgm2 : Outport  Port=3
  spd_in_radps : Outport  Port=4
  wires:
  gearbox/1(bus_out) -> Bus Creator/1  "gearbox"
  gearbox/2(trq_out_Nm) -> trq_out_Nm/1
  gearbox/3(iner_out_kgm2) -> iner_out_kgm2/1
  gearbox/4(spd_in_radps) -> spd_in_radps/1, Bus Creator/2  "trans_spd_in_radps"
  trans_bus/1 -> gearbox/1(trans_bus)
  Bus Creator/1 -> bus_out/1  "trans"
  spd_out_radps/1 -> gearbox/4(spd_out_radps), Bus Creator/3  "trans_spd_out_radps"
  iner_in_kgm2/1 -> gearbox/3(iner_in_kgm2)
  trq_in_Nm/1 -> gearbox/2(trq_in_Nm)

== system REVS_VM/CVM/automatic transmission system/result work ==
  torque_Nm : Inport
  speed_radps : Inport  Port=2
  upstream_iner_kgm2 : Inport  Port=3
  Derivative : Derivative  CoefficientInTFapproximation=1e6
  Gain : Gain  Gain=1/1000
  Integrator1 : Integrator  UpperSaturationLimit=Inf  LowerSaturationLimit=0  ZeroCross=off
  Integrator2 : Integrator  UpperSaturationLimit=Inf  LowerSaturationLimit=0  ZeroCross=off
  Phase To Workspace : ToWorkspace  VariableName=result__phase_transmission_output_pos_work_kJ  SampleTime=-1
  Pos : Fcn  Expr=u(1)*(u(1) >= 0)
  Product : Product
  Product1 : Product
  Product2 : Product
  Subtract : Sum  Inputs=+-
  Total To Workspace : ToWorkspace  VariableName=result__total_transmission_output_pos_work_kJ  SampleTime=-1
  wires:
  Product2/1 -> Pos/1
  Pos/1 -> Gain/1
  Gain/1 -> Integrator1/1, Product/2
  Product1/1 -> Subtract/2
  Derivative/1 -> Product1/1
  speed_radps/1 -> Derivative/1, Product2/2
  upstream_iner_kgm2/1 -> Product1/2
  Subtract/1 -> Product2/1
  Integrator2/1 -> Phase To Workspace/1
  [REVS_phase_flag] -> Product/1
  Product/1 -> Integrator2/1
  Integrator1/1 -> Total To Workspace/1
  torque_Nm/1 -> Subtract/1

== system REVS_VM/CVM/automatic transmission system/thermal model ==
  note: 1) Only subsystems can be added as variant choices at this level 2) Blocks cannot be connected at this level as connectivity is automatically determined at simulation, based on the active variant
  system_bus : Inport
  constant temperature : Subsystem  VariantControl="get_REVS_transmission_thermal_type( transmission) ==  enum_transmission_thermal_type.constant_temperature"
  gradient warmup : Subsystem  VariantControl=get_REVS_transmission_thermal_type( transmission) == enum_transmission_thermal_type.gradient_temperature
  none : Subsystem  VariantControl="get_REVS_transmission_thermal_type( transmission) ==  enum_transmission_thermal_type.none"
  thermal model : Subsystem  VariantControl="get_REVS_transmission_thermal_type( transmission) ==  enum_transmission_thermal_type.thermal_model"
  time lookup : Subsystem  VariantControl="get_REVS_transmission_thermal_type( transmission) ==  enum_transmission_thermal_type.time_lookup"
  thermal_bus : Outport

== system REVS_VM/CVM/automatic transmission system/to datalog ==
  Var : Inport
  Constant : Constant  Value=VerboseSignal
  Constant1 : Constant  Value=VerboseLevel
  Relational Operator : RelationalOperator  OutDataTypeStr=boolean  ZeroCross=off
  Subsystem : Subsystem
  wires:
  Constant1/1 -> Relational Operator/2
  Constant/1 -> Relational Operator/1
  Relational Operator/1 -> Subsystem/Enable
  Var/1 -> Subsystem/1(In1)

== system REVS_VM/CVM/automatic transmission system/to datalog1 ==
  Var : Inport
  Constant : Constant  Value=VerboseSignal
  Constant1 : Constant  Value=VerboseLevel
  Relational Operator : RelationalOperator  OutDataTypeStr=boolean  ZeroCross=off
  Subsystem : Subsystem
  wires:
  Constant1/1 -> Relational Operator/2
  Constant/1 -> Relational Operator/1
  Relational Operator/1 -> Subsystem/Enable
  Var/1 -> Subsystem/1(In1)

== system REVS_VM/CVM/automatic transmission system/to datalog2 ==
  Var : Inport
  Constant : Constant  Value=VerboseSignal
  Constant1 : Constant  Value=VerboseLevel
  Relational Operator : RelationalOperator  OutDataTypeStr=boolean  ZeroCross=off
  Subsystem : Subsystem
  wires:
  Constant1/1 -> Relational Operator/2
  Constant/1 -> Relational Operator/1
  Relational Operator/1 -> Subsystem/Enable
  Var/1 -> Subsystem/1(In1)

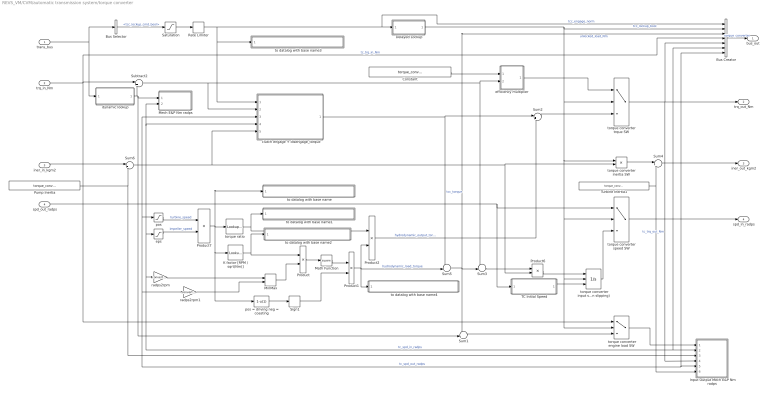
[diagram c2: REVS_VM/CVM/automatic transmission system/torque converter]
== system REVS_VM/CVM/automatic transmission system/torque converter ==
  trans_bus : Inport
  trq_in_Nm : Inport  Port=2
  iner_in_kgm2 : Inport  Port=3
  spd_out_radps : Inport  Port=4
  " torque converter engine load SW" : Switch  Threshold=0.5
  " torque converter input speed integrator (integrate when slipping)" : Integrator  ExternalReset=falling  InitialConditionSource=external  LimitOutput=on  UpperSaturationLimit=Inf  LowerSaturationLimit=0
  Bus Selector : BusSelector  OutputSignals=ctrl.tcc_lockup_cmd_bool
  Bus Creator : BusCreator  Inputs=7
  Constant : Constant  Value=torque_converter.lockup_efficiency_norm
  Delayed Lockup : Subsystem
  Input Output Mech E&P Nm radps : Subsystem
  K factor [RPM / sqrt(Nm)] : Lookup_n-D  NumberOfTableDimensions=1  BreakpointsForDimension1=torque_converter.all_speed_ratios  IndexSearchMethod=Linear search  BeginIndexSearchUsingPreviousIndexResult=on  Table=torque_converter.all_k_factors_rpmpsqrtNm  ExtrapMethod=Clip  UseLastTableValue=on  InternalRulePriority=Speed  RndMeth=Simplest
  Math Function : Math  Operator=square
  Mech E&P Nm radps : Subsystem
  MinMax : MinMax  Function=max  Inputs=2  ZeroCross=off
  Product : Product  Inputs=/*
  Product1 : Product
  Product2 : Product
  Product6 : Product  Inputs=*/
  Product7 : Product  Inputs=*/
  Pump Inertia : Constant  Value=torque_converter.pump_inertia_kgm2
  Rate Limiter : RateLimiter  RisingSlewLimit=1/torque_converter.lockup_duration_secs  FallingSlewLimit=-1/torque_converter.unlock_duration_secs  InitialCondition=1
  Saturation : Saturate  UpperLimit=1  LowerLimit=0
  Sign1 : Signum  ZeroCross=off
  Subtract2 : Sum  Inputs=|+-
  Sum1 : Sum  Inputs=++|
  Sum2 : Sum  Inputs=|++
  Sum3 : Sum  Inputs=+-|
  Sum4 : Sum  Inputs=|++
  Sum5 : Sum  Inputs=++|
  Sum6 : Sum  Inputs=|++
  TC Initial Speed : Subsystem
  Turbine Inertia1 : Constant  Value=torque_converter.turbine_inertia_kgm2
  clutch engage + disengage_torque : Subsystem
  dynamic lookup : Subsystem
  efficiency multiplier : Subsystem
  eps : Saturate  UpperLimit=inf  LowerLimit=eps
  pos : Saturate  UpperLimit=inf  LowerLimit=0
  pos = driving neg = coasting : Fcn  Expr=1-u(1)
  radps2rpm : Gain  Gain=convert.radps2rpm
  radps2rpm1 : Gain  Gain=convert.radps2rpm
  to datalog with base name : Subsystem
  to datalog with base name1 : Subsystem
  to datalog with base name2 : Subsystem
  to datalog with base name3 : Subsystem
  to datalog with base name4 : Subsystem
  torque converter inertia SW : Product
  torque converter trque SW : Switch  Threshold=0.5
  torque converter speed SW : Switch  Threshold=0.5
  torque ratio : Lookup_n-D  NumberOfTableDimensions=1  BreakpointsForDimension1=torque_converter.all_speed_ratios  IndexSearchMethod=Linear search  BeginIndexSearchUsingPreviousIndexResult=on  Table=torque_converter.all_torque_ratios  ExtrapMethod=Clip  UseLastTableValue=on  InternalRulePriority=Speed  RndMeth=Simplest
  bus_out : Outport
  trq_out_Nm : Outport  Port=2
  iner_out_kgm2 : Outport  Port=3
  spd_in_radps : Outport  Port=4
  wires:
  efficiency multiplier/1(output) -> torque converter trque SW/1
  Constant/1 -> efficiency multiplier/1(efficiency)
  trq_in_Nm/1 -> " torque converter engine load SW"/1, Bus Creator/4, Subtract2/1  "tc_trq_in_Nm"
  spd_out_radps/1 -> TC Initial Speed/1(In), torque converter speed SW/1, clutch engage + disengage_torque/3(final_spd_radps), pos/1, Bus Creator/7, Input Output Mech E&P Nm radps/5(spd_out_radps), radps2rpm1/1  "tc_spd_out_radps"
  trans_bus/1 -> dynamic lookup/1(bus), Bus Selector/1
  Rate Limiter/1 -> clutch engage + disengage_torque/1(engage), to datalog with base name3/1(Var), Delayed Lockup/1(Engage), Bus Creator/1  "tcc_engage_norm"
  Sum5/1 -> Bus Creator/3, Sum3/2, Sum1/1  "unlocked_load_Nm"
  Bus Creator/1 -> bus_out/1  "torque_converter"
  pos/1 -> Product7/1  "turbine_speed"
  eps/1 -> Product7/2  "impeller_speed"
  Delayed Lockup/1(Lockup) -> Bus Creator/2, torque converter trque SW/2, torque converter inertia SW/1, torque converter speed SW/2, " torque converter input speed integrator (integrate when slipping)"/2, " torque converter engine load SW"/2  "tcc_lockup_bool"
  Product2/1 -> Sum2/2  "hydrodynamic_output_torque"
  Sum2/1 -> torque converter trque SW/3
  clutch engage + disengage_torque/1(tcc_torque_Nm) -> Sum5/1, Sum2/1  "tcc_torque"
  Sum6/1 -> torque converter inertia SW/2, Product6/2, clutch engage + disengage_torque/5(iner_in_kgm2)
  Bus Selector/1 -> Saturation/1  "<tcc_lockup_cmd_bool>"
  iner_in_kgm2/1 -> Sum6/1
  TC Initial Speed/1(Out) -> " torque converter input speed integrator (integrate when slipping)"/3
  Product6/1 -> " torque converter input speed integrator (integrate when slipping)"/1
  Sum1/1 -> " torque converter engine load SW"/3
  " torque converter engine load SW"/1 -> Input Output Mech E&P Nm radps/1(trq_in_Nm)
  Product7/1 -> pos = driving neg = coasting/1, K factor [RPM / sqrt(Nm)]/1, to datalog with base name/1(Var), torque ratio/1
  K factor [RPM / sqrt(Nm)]/1 -> Product/1, to datalog with base name2/1(Var)
  torque converter speed SW/1 -> spd_in_radps/1, Bus Creator/6, eps/1, Mech E&P Nm radps/2(spd_radps), clutch engage + disengage_torque/4(current_spd_radps), radps2rpm/1, Input Output Mech E&P Nm radps/2(spd_in_radps)  "tc_spd_in_radps"
  Subtract2/1 -> Sum3/1, efficiency multiplier/2(input), clutch engage + disengage_torque/2(trq_in_Nm)
  Product/1 -> Math Function/1
  Math Function/1 -> Product1/1
  pos = driving neg = coasting/1 -> Sign1/1
  radps2rpm/1 -> MinMax/1
  radps2rpm1/1 -> MinMax/2
  Product1/1 -> Product2/2, Sum5/2, to datalog with base name4/1(Var)  "hydrodynamic_load_torque"
  Sign1/1 -> Product1/2
  " torque converter input speed integrator (integrate when slipping)"/1 -> torque converter speed SW/3
  torque converter trque SW/1 -> Bus Creator/5, Input Output Mech E&P Nm radps/4(trq_out_Nm), trq_out_Nm/1  "tc_trq_out_Nm"
  torque converter inertia SW/1 -> Sum4/1
  Sum3/1 -> Product6/1
  Sum4/1 -> iner_out_kgm2/1
  torque ratio/1 -> Product2/1, to datalog with base name1/1(Var)
  Pump Inertia/1 -> Sum6/2, Input Output Mech E&P Nm radps/3(iner_in_kgm2)
  Turbine Inertia1/1 -> Sum4/2, Input Output Mech E&P Nm radps/6(iner_out_kgm2)
  dynamic lookup/1(out) -> Mech E&P Nm radps/1(trq_Nm), Sum1/2, Subtract2/2
  MinMax/1 -> Product/2
  Saturation/1 -> Rate Limiter/1
